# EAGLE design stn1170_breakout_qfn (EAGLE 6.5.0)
DESCRIPTION: Breakout Board; HW_REV: 1.1; PCB_REV: B; TITLE: STN1170 - Breakout Board

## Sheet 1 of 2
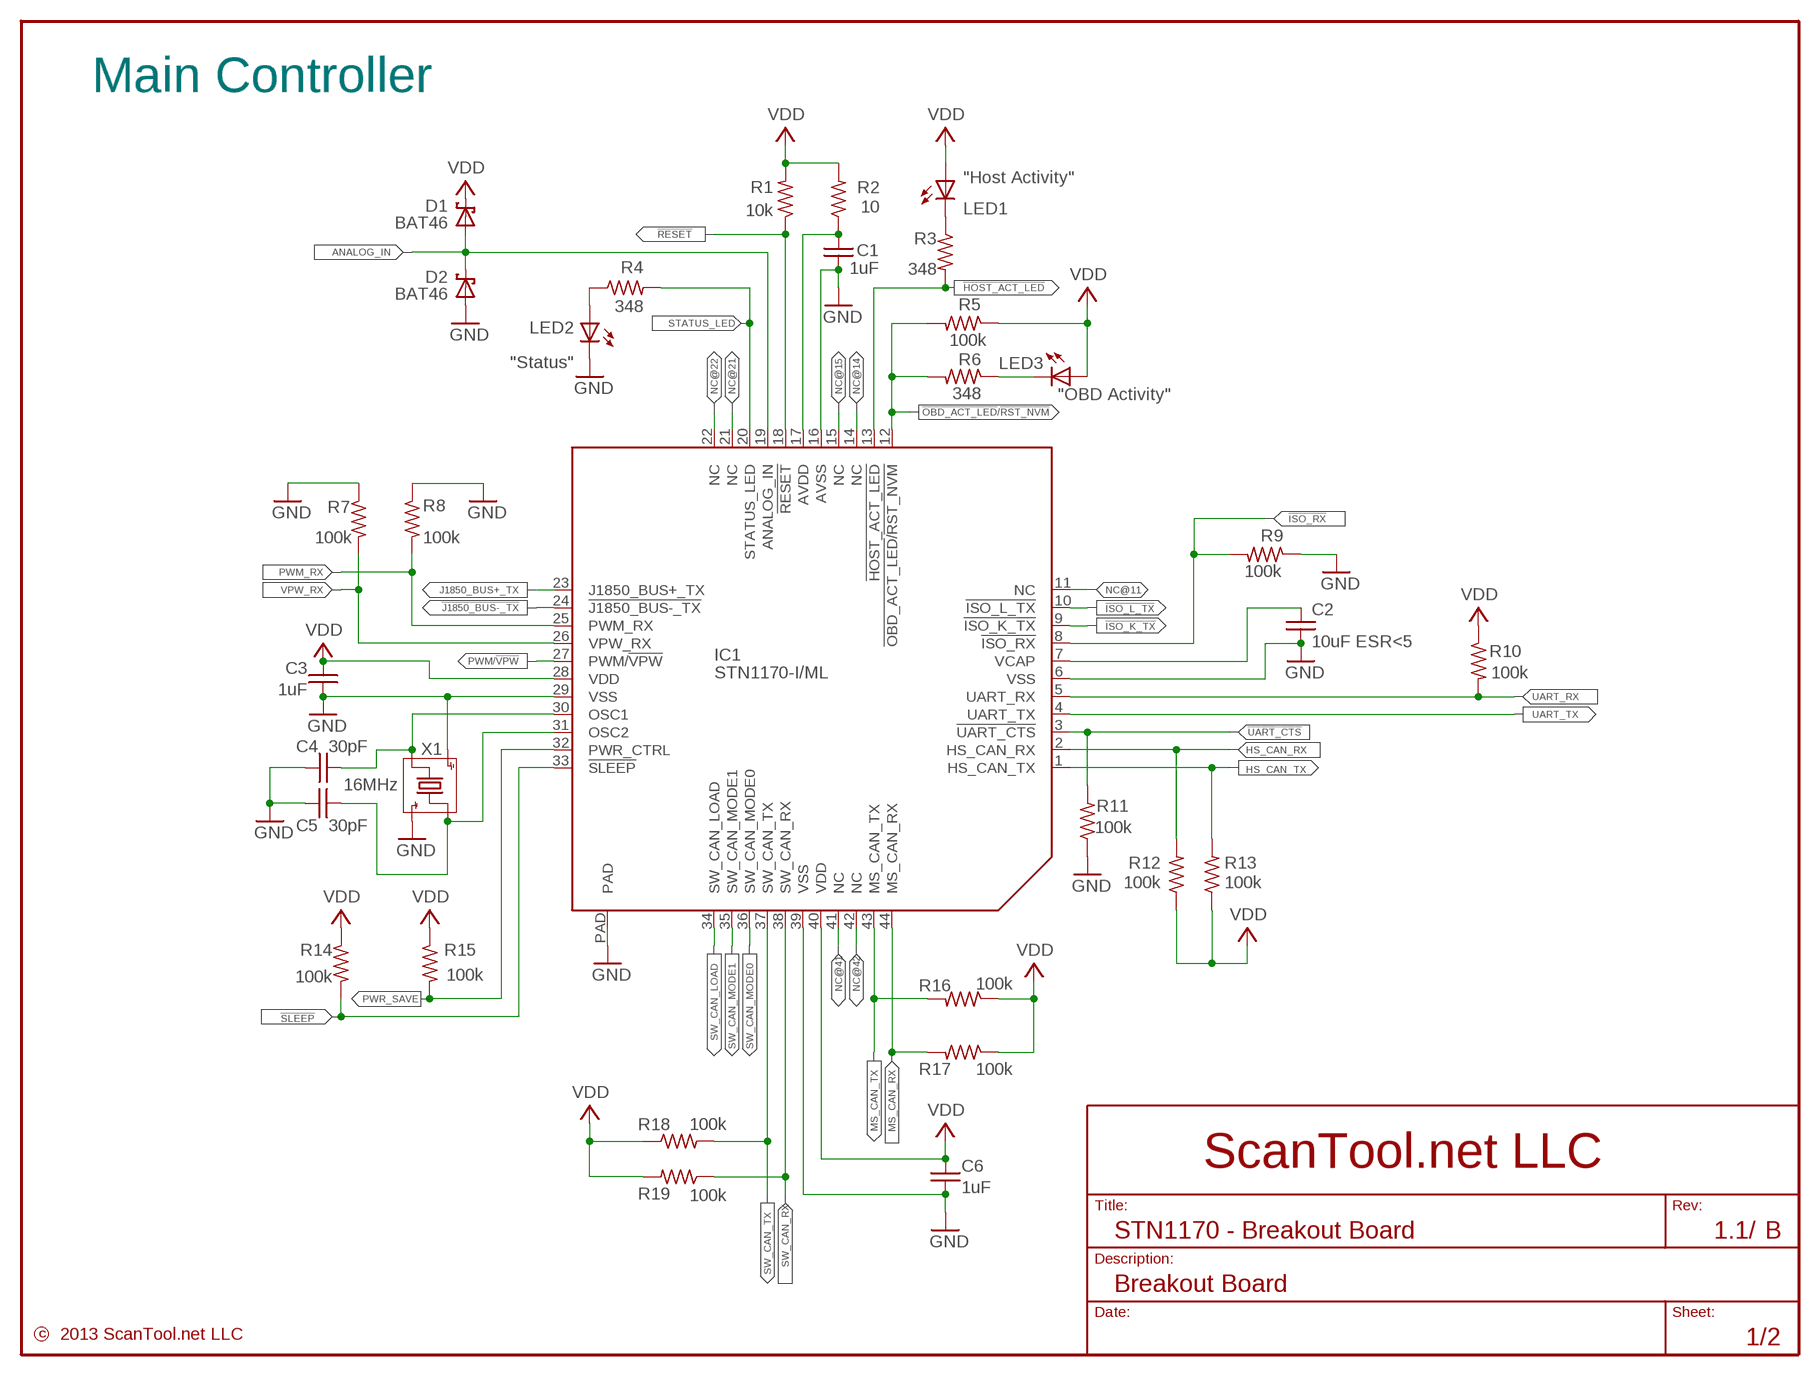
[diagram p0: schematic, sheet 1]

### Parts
C1  1uF  C-US_0603  [0603]
C2  10uF ESR<5  C-US_0805  [0805]
C3  1uF  C-US_0603  [0603]
C4  30pF  C-US_0603  [0603]
C5  30pF  C-US_0603  [0603]
C6  1uF  C-US_0603  [0603]
D1  BAT46  BAT46JFILM  [SOD-323_SCHOTTKY]
D2  BAT46  BAT46JFILM  [SOD-323_SCHOTTKY]
IC1  STN1170-I/ML  [QFN-44]
LED1  "Host Activity"  LED-0805  [0805-LED]
LED2  "Status"  LED-0805  [0805-LED]
LED3  "OBD Activity"  LED-0805  [0805-LED]
R1  10k  R-US_0603  [0603]
R2  10  R-US_0603  [0603]
R3  348  R-US_0603  [0603]
R4  348  R-US_0603  [0603]
R5  100k  R-US_0603  [0603]
R6  348  R-US_0603  [0603]
R7  100k  R-US_0603  [0603]
R8  100k  R-US_0603  [0603]
R9  100k  R-US_0603  [0603]
R10  100k  R-US_0603  [0603]
R11  100k  R-US_0603  [0603]
R12  100k  R-US_0603  [0603]
R13  100k  R-US_0603  [0603]
R14  100k  R-US_0603  [0603]
R15  100k  R-US_0603  [0603]
R16  100k  R-US_0603  [0603]
R17  100k  R-US_0603  [0603]
R18  100k  R-US_0603  [0603]
R19  100k  R-US_0603  [0603]
X1  16MHz  CRYSTAL-4PIN_NX3225SA  [3.2X2.5-MM]

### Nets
!HOST_ACT_LED: IC1.13(!HOST_ACT_LED) R3.2 ; also sheet 2
!ISO_K_TX: IC1.9(!ISO_K_TX) ; also sheet 2
!ISO_L_TX: IC1.10(!ISO_L_TX) ; also sheet 2
!ISO_RX: IC1.8(!ISO_RX) R9.2 ; also sheet 2
!J1850_BUS-_TX: IC1.24(!J1850_BUS-_TX) ; also sheet 2
!OBD_ACT_LED!/!RST_NVM: IC1.12(!OBD_ACT_LED!/!RST_NVM) R5.2 R6.2 ; also sheet 2
!RESET: IC1.18(!RESET) R1.1 ; also sheet 2
!SLEEP: IC1.33(!SLEEP) R14.2 ; also sheet 2
!UART_CTS: IC1.3(!UART_CTS) R11.2 ; also sheet 2
ANALOG_IN: D1.A D2.C IC1.19(ANALOG_IN) ; also sheet 2
AVDD [Supply]: C1.1 IC1.17(AVDD) R2.1
GND [Supply]: C1.2 C2.2 C3.1 C4.2 C5.2 C6.2 D2.A IC1.6(VSS) IC1.16(AVSS) IC1.29(VSS) IC1.39(VSS) IC1.PAD LED2.C R7.1 R8.1 R9.1 R11.1 X1.2(GND) X1.4(GND) ; also sheet 2
HS_CAN_RX: IC1.2(HS_CAN_RX) R12.2 ; also sheet 2
HS_CAN_TX: IC1.1(HS_CAN_TX) R13.2 ; also sheet 2
J1850_BUS+_TX: IC1.23(J1850_BUS+_TX) ; also sheet 2
MS_CAN_RX: IC1.44(MS_CAN_RX) R17.2 ; also sheet 2
MS_CAN_TX: IC1.43(MS_CAN_TX) R16.2 ; also sheet 2
N$1: LED1.C R3.1
N$2: LED3.C R6.1
N$3: C5.1 IC1.31(OSC2) X1.1(OSCX)
N$4: LED2.A R4.1
N$6: C4.1 IC1.30(OSC1) X1.3(OSCX)
NC@11: IC1.11(NC) ; also sheet 2
NC@14: IC1.14(NC) ; also sheet 2
NC@15: IC1.15(NC) ; also sheet 2
NC@21: IC1.21(NC) ; also sheet 2
NC@22: IC1.22(NC) ; also sheet 2
NC@41: IC1.41(NC) ; also sheet 2
NC@42: IC1.42(NC) ; also sheet 2
PWM/!VPW: IC1.27(PWM/!VPW) ; also sheet 2
PWM_RX: IC1.25(PWM_RX) R8.2 ; also sheet 2
PWR_SAVE: IC1.32(PWR_CTRL) R15.2 ; also sheet 2
STATUS_LED: IC1.20(STATUS_LED) R4.2 ; also sheet 2
STN1170_VCAP: C2.1 IC1.7(VCAP)
SW_CAN_LOAD: IC1.34(SW_CAN_LOAD) ; also sheet 2
SW_CAN_MODE0: IC1.36(SW_CAN_MODE0) ; also sheet 2
SW_CAN_MODE1: IC1.35(SW_CAN_MODE1) ; also sheet 2
SW_CAN_RX: IC1.38(SW_CAN_RX) R19.1 ; also sheet 2
SW_CAN_TX: IC1.37(SW_CAN_TX) R18.2 ; also sheet 2
UART_RX: IC1.5(UART_RX) R10.2 ; also sheet 2
UART_TX: IC1.4(UART_TX) ; also sheet 2
VDD [Supply]: C3.2 C6.1 D1.C IC1.28(VDD) IC1.40(VDD) LED1.A LED3.A R1.2 R2.2 R5.1 R10.1 R12.1 R13.1 R14.1 R15.1 R16.1 R17.1 R18.1 R19.2 ; also sheet 2
VPW_RX: IC1.26(VPW_RX) R7.2 ; also sheet 2

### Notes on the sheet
- Main Controller
- BAT46
- BAT46

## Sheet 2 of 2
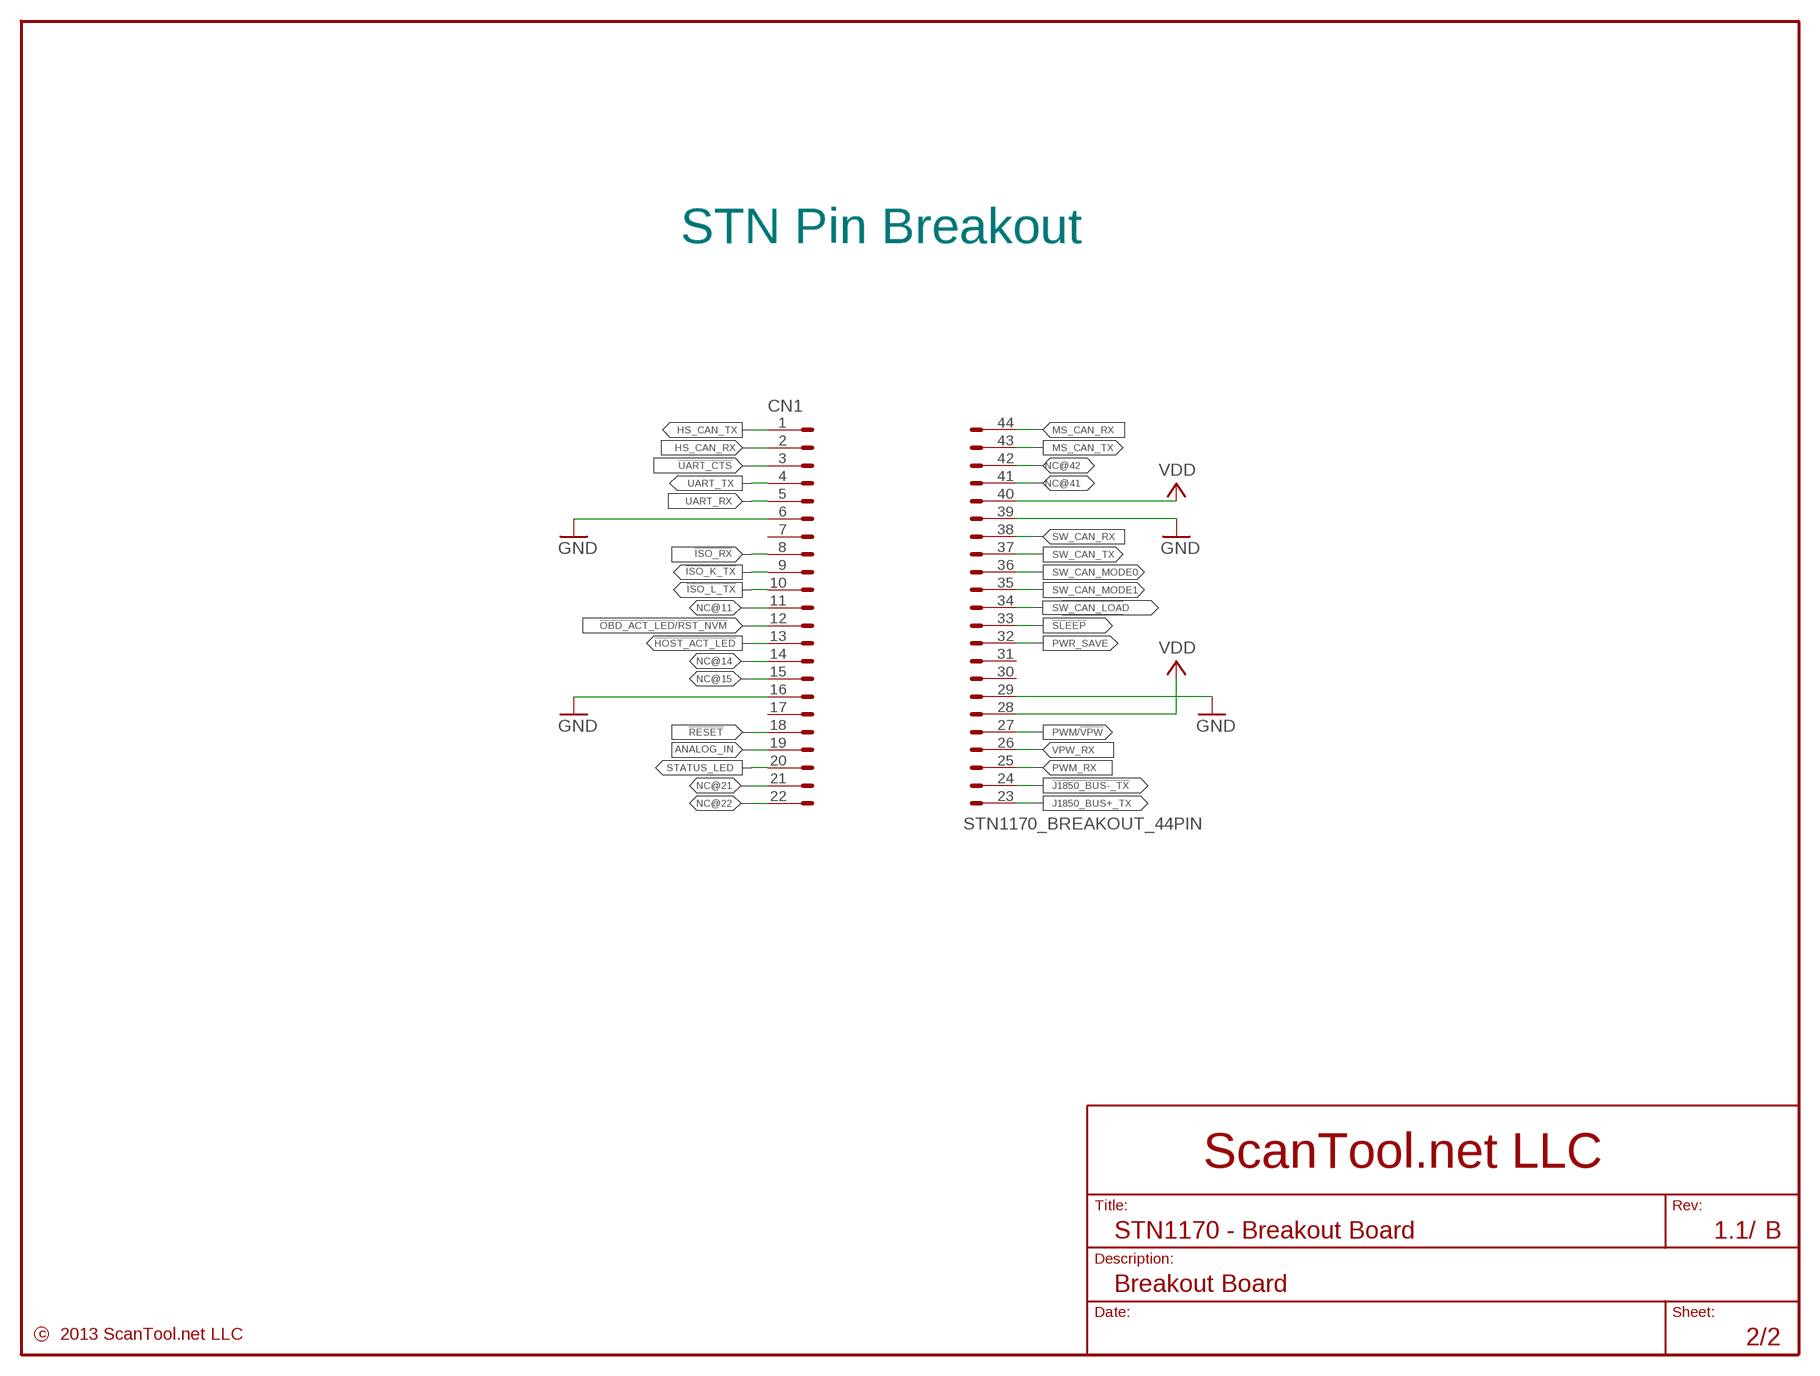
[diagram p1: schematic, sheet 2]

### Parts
CN1  STN1170_BREAKOUT_44PIN  [STN1170_BREAKOUT_44PIN]

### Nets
!HOST_ACT_LED: CN1.13 ; also sheet 1
!ISO_K_TX: CN1.9 ; also sheet 1
!ISO_L_TX: CN1.10 ; also sheet 1
!ISO_RX: CN1.8 ; also sheet 1
!J1850_BUS-_TX: CN1.24 ; also sheet 1
!OBD_ACT_LED!/!RST_NVM: CN1.12 ; also sheet 1
!RESET: CN1.18 ; also sheet 1
!SLEEP: CN1.33 ; also sheet 1
!UART_CTS: CN1.3 ; also sheet 1
ANALOG_IN: CN1.19 ; also sheet 1
GND [Supply]: CN1.6 CN1.16 CN1.29 CN1.39 ; also sheet 1
HS_CAN_RX: CN1.2 ; also sheet 1
HS_CAN_TX: CN1.1 ; also sheet 1
J1850_BUS+_TX: CN1.23 ; also sheet 1
MS_CAN_RX: CN1.44 ; also sheet 1
MS_CAN_TX: CN1.43 ; also sheet 1
NC@11: CN1.11 ; also sheet 1
NC@14: CN1.14 ; also sheet 1
NC@15: CN1.15 ; also sheet 1
NC@21: CN1.21 ; also sheet 1
NC@22: CN1.22 ; also sheet 1
NC@41: CN1.41 ; also sheet 1
NC@42: CN1.42 ; also sheet 1
PWM/!VPW: CN1.27 ; also sheet 1
PWM_RX: CN1.25 ; also sheet 1
PWR_SAVE: CN1.32 ; also sheet 1
STATUS_LED: CN1.20 ; also sheet 1
SW_CAN_LOAD: CN1.34 ; also sheet 1
SW_CAN_MODE0: CN1.36 ; also sheet 1
SW_CAN_MODE1: CN1.35 ; also sheet 1
SW_CAN_RX: CN1.38 ; also sheet 1
SW_CAN_TX: CN1.37 ; also sheet 1
UART_RX: CN1.5 ; also sheet 1
UART_TX: CN1.4 ; also sheet 1
VDD [Supply]: CN1.28 CN1.40 ; also sheet 1
VPW_RX: CN1.26 ; also sheet 1
Unconnected: CN1.7 CN1.17 CN1.30 CN1.31

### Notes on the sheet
- STN Pin Breakout

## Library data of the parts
C1-C6 = _stn_rcl:C-US: Capacitor, US Symbol; DESC: Capacitor; VALSTAT: VAL
CN1 = _stn_connector:STN1170_BREAKOUT_44PIN: STN1170-BREAKOUT BOARD, Male, 22X2, .0.01" Pitch Based on 2 Standard 22X1 .01" pitch male headers. Change Log DateAuthorChange July 05, 2012dduggan@scantool.netDevice created.; DESC: Header; PARTNUM: 0.1" male header; VALSTAT: PARTNUM
D1 D2 = _stn_diode:BAT46?FILM: BAT46 Schottky Diode; DESC: Diode, Schottky; MANUF: STMicroelectronics; PARTNUM: BAT46JFILM; SUPPLIER: Digikey:497-6653-1-ND; VALSTAT: PARTNUM
IC1 = _stn_scantool:STN1170: STN1170 Change Log DateAuthorChange July 12, 2012jason@scantool.netAdded attributes to device July 11, 2012vitaliy@scantool.netRenamed SW_CAN_HS_MODE pin to SW_CAN_LOAD April 11, 2012vit@scantool.netChanged UART_CTS pin polarity. Renamed OSCI/OSCOpins to OSC1/OSC2. April 10,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; DESC: IC, OBD-to-UART; MANUF: ScanTool.net, LLC; PARTNUM: ???; VALSTAT: VALUE
LED1-LED3 = _stn_led:LED: Light Emitting Diode; DESC: LED; VALSTAT: LABEL
R1-R19 = _stn_rcl:R-US: Resistor, US Symbol; DESC: Resistor; VALSTAT: VAL
X1 = _stn_crystal:CRYSTAL-4PIN: Crystal, 4 PIN March 16, 2010 vitaliy@scantool.netFixed pin assignments, verified package. March 4, 2010 jason@scantool.netCreated device from the NDK NX3225SA datasheet.; DESC: Crystal; MANUF: TXC; PARTNUM: 7M; VALSTAT: VAL

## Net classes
0 default: width 0.203 mm, drill 0.406 mm, clearance 0.203 mm
1 Supply: width 0.305 mm, drill 0.508 mm, clearance 0.254 mm
2 Vbat: width 0.61 mm, drill 0.813 mm, clearance 0.381 mm

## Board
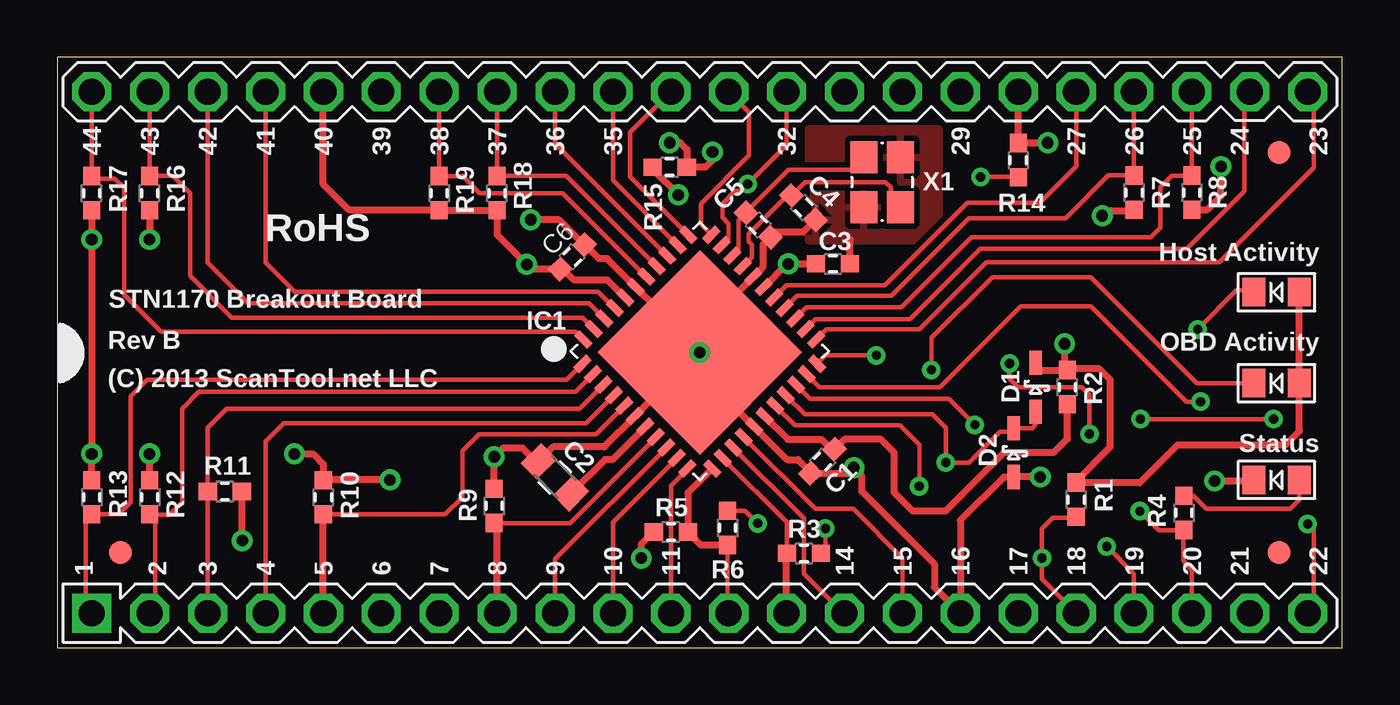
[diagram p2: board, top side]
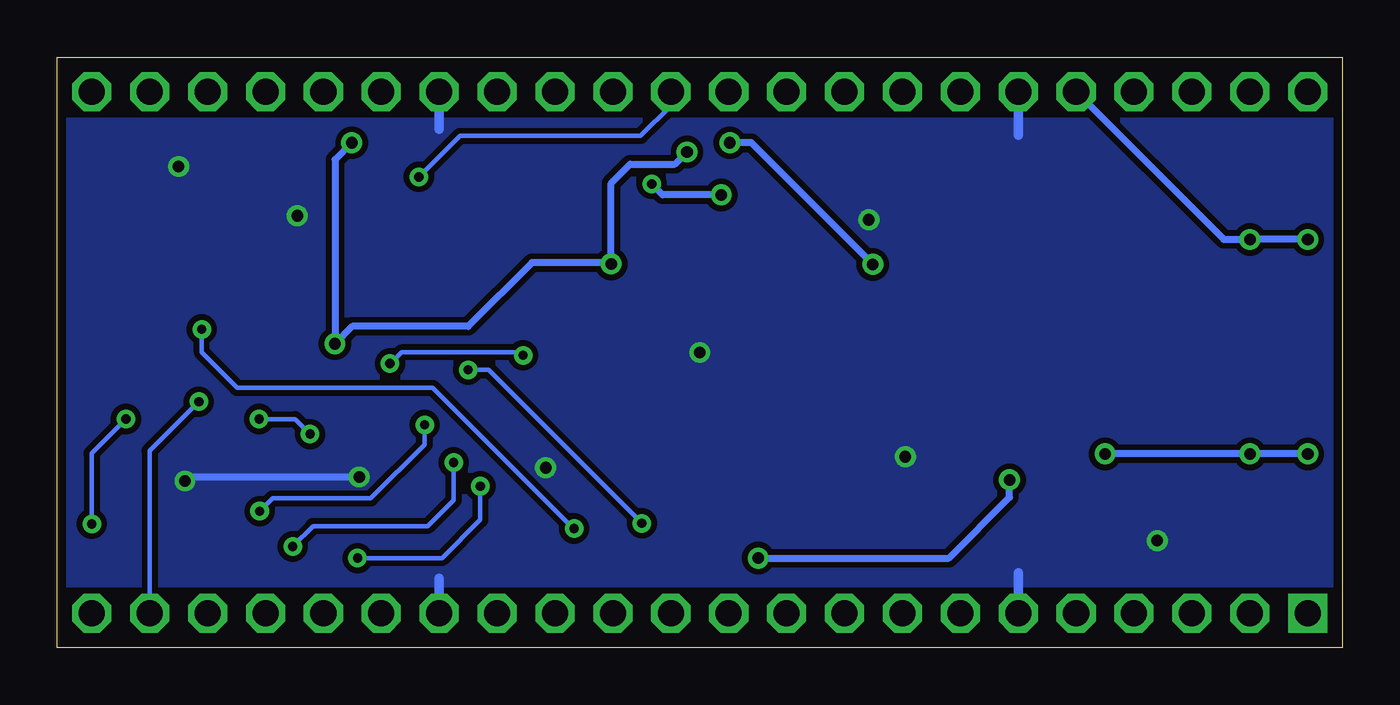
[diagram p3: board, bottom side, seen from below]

Size 56.39 x 25.91 mm. Coordinates in mm from the lower left corner, seen from the top.
Outline: 56.39,0 56.39,25.91 0,25.91 0,0 56.39,0
Copper layers (1*16): Top 0.035mm / dielectric 1.5mm / Bottom 0.035mm
Design rules "default": minimum track width 8mil, minimum drill 15mil, track to track 8mil, track to pad 8mil, pad to pad 8mil, via to via 8mil, smd to smd 8mil, copper to edge 15mil, drill to drill 8mil, minimum pad ring 10mil, minimum via ring 8mil, stop-mask expansion 4mil, vias tented up to drill 20mil, thermal gap 10mil

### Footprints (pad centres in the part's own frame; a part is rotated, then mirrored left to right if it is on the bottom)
0603 = smd 0.8 x 0.75: 1 -0.75,0; 2 0.75,0
0805 = smd 1 x 1.25: 1 -1,0; 2 1,0
STN1170_BREAKOUT_44PIN = drill 1.143 square: 1 -11.43,26.67 | drill 1.143 octagon: 2 -11.43,24.13; 3 -11.43,21.59; 4 -11.43,19.05; 5 -11.43,16.51; 6 -11.43,13.97; 7 -11.43,11.43; 8 -11.43,8.89; 9 -11.43,6.35; 10 -11.43,3.81; 11 -11.43,1.27; 12 -11.43,-1.27; 13 -11.43,-3.81; 14 -11.43,-6.35; 15 -11.43,-8.89; 16 -11.43,-11.43; 17 -11.43,-13.97; 18 -11.43,-16.51; 19 -11.43,-19.05; 20 -11.43,-21.59; 21 -11.43,-24.13; 22 -11.43,-26.67; 23 11.43,-26.67; 24 11.43,-24.13; 25 11.43,-21.59; 26 11.43,-19.05; 27 11.43,-16.51; 28 11.43,-13.97; 29 11.43,-11.43; 30 11.43,-8.89; 31 11.43,-6.35; 32 11.43,-3.81; 33 11.43,-1.27; 34 11.43,1.27; 35 11.43,3.81; 36 11.43,6.35; 37 11.43,8.89; 38 11.43,11.43; 39 11.43,13.97; 40 11.43,16.51; 41 11.43,19.05; 42 11.43,21.59; 43 11.43,24.13; 44 11.43,26.67
SOD-323_SCHOTTKY = smd 1.06 x 0.54: A 1.07,0; C -1.07,0
FIDUCIAL_40X100 = smd 1.016 x 1.016: P$1 0,0
QFN-44 = smd 0.8 x 0.35: 1 -3.988,3.287; 2 -3.988,2.637; 3 -3.988,1.987; 4 -3.988,1.337; 5 -3.988,0.687; 6 -3.988,0.037; 7 -3.988,-0.613; 8 -3.988,-1.263; 9 -3.988,-1.913; 10 -3.988,-2.563; 11 -3.988,-3.213; 23 4.012,-3.213; 24 4.012,-2.563; 25 4.012,-1.913; 26 4.012,-1.263; 27 4.012,-0.613; 28 4.012,0.037; 29 4.012,0.687; 30 4.012,1.337; 31 4.012,1.987; 32 4.012,2.637; 33 4.012,3.287 | smd 0.35 x 0.8: 12 -3.213,-3.988; 13 -2.563,-3.988; 14 -1.913,-3.988; 15 -1.263,-3.988; 16 -0.613,-3.988; 17 0.037,-3.988; 18 0.687,-3.988; 19 1.337,-3.988; 20 1.987,-3.988; 21 2.637,-3.988; 22 3.287,-3.988; 34 3.287,4.012; 35 2.637,4.012; 36 1.987,4.012; 37 1.337,4.012; 38 0.687,4.012; 39 0.037,4.012; 40 -0.613,4.012; 41 -1.263,4.012; 42 -1.913,4.012; 43 -2.563,4.012; 44 -3.213,4.012 | smd 6.35 x 6.35: PAD 0,0
0805-LED = smd 1 x 1.25: A 1,0; C -1,0
3.2X2.5-MM = smd 1.4 x 1.2: 1 -1.1,-0.8; 2 1.1,-0.8; 3 1.1,0.8; 4 -1.1,0.8

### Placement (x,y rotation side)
C1  33.58,8.18 225 top
C2  21.84,7.48 135 top
C3  34.04,16.84 180 top
C4  32.75,19.31 315 top
C5  30.76,18.54 315 top
C6  22.6,17.14 45 top
CN1  28.19,12.95 90 top
D1  42.93,11.43 270 top
D2  41.96,8.56 270 top
E$4  [FIDUCIAL_40X100]  53.59,21.72 0 top
E$5  [FIDUCIAL_40X100]  2.79,4.19 0 top
E$6  [FIDUCIAL_40X100]  53.59,4.19 180 top
IC1  28.19,12.95 45 top
LED1  53.49,15.6 0 top
LED2  53.49,7.37 0 top
LED3  53.49,11.61 0 top
R1  44.7,6.5 90 top
R2  44.32,11.43 90 top
R3  32.77,4.14 180 top
R4  49.43,5.92 270 top
R5  26.92,5.08 0 top
R6  29.41,5.26 270 top
R7  47.24,19.96 90 top
R8  49.78,19.96 90 top
R9  19.18,6.22 270 top
R10  11.68,6.6 270 top
R11  7.37,6.86 180 top
R12  4.06,6.6 270 top
R13  1.52,6.6 270 top
R14  42.16,21.39 270 top
R15  26.87,21.08 180 top
R16  4.06,19.94 90 top
R17  1.52,19.94 90 top
R18  19.3,19.94 90 top
R19  16.76,19.94 270 top
X1  36.2,20.42 270 top

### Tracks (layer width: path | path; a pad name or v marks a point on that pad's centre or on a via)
!HOST_ACT_LED
  Top 0.203: R3.2 32.02,5.51 IC1.13
  Top 0.305: CN1.13 32,4.13 R3.2
!ISO_K_TX
  Top 0.203: IC1.9 21.84,3.9 CN1.9
!ISO_L_TX
  Top 0.203: IC1.10 24.38,5.51 CN1.10
!ISO_RX
  Top 0.203: IC1.8 22.5,5.47 R9.2
  Top 0.305: CN1.8 19.3,5.35 R9.2
!J1850_BUS-_TX
  Top 0.203: IC1.24 33.27,14.4 37.41,14.4 40.51,17.5 49.55,17.5 52.07,20.02 52.07,24.13 CN1.24
!OBD_ACT_LED!/!RST_NVM
  Top 0.203: R6.2 29.41,1.57 CN1.12
  Top 0.305: IC1.12 27.67,6.79 R5.2 28.25,4.51 R6.2
!RESET  (via drill 0.41)
  Top 0.203: R1.1 44.67,5.71 43.69,5.71 43.2,5.23 v43.2,3.94 43.2,3.02 CN1.18 | IC1.18 32.37,9.75 36.98,9.75 37.82,8.91 v37.82,7.09
  Bottom 0.203: v37.82,7.09 37.82,5.61 39.5,3.94 v43.2,3.94
!SLEEP  (via drill 0.41)
  Top 0.203: R14.2 v40.51,20.65 | IC1.33 28.25,18.58 28.25,19.48 30.35,21.59 30.35,23.5 CN1.33 29.48,24.38
  Bottom 0.203: v40.51,20.65 38.71,22.45 30.79,22.45 29.46,23.77 CN1.33
!UART_CTS
  Top 0.203: IC1.3 22.92,10.49 7.44,10.49 6.6,9.65 6.6,6.87 | 6.6,6.87 R11.2 | 6.6,6.87 CN1.3
ANALOG_IN  (via drill 0.41)
  Top 0.203: IC1.19 32.8,10.24 38.41,10.24 38.99,9.65 v38.99,8.13 40.01,8.13 41.35,9.47 41.8,9.47 D2.C 42.78,9.63 42.93,9.78 D1.A | CN1.19 47.24,3.25 v46.05,4.45
  Bottom 0.203: v38.99,8.13 38.99,6.48 40.13,5.33 45.16,5.33 v46.05,4.45
AVDD
  Top 0.305: IC1.17 32.06,9.14 33.53,9.14 33.96,8.71 C1.1 34.54,9.14 36.14,9.14 36.73,8.56 36.73,6.81 37.54,5.99 38.96,5.99 41.53,8.56 43.71,8.56 44.32,9.17 R2.1
GND  (via drill 0.51)
  Top 0.305: X1.4 36.99,21.73 | v43.13,7.49 41.99,7.49 41.98,7.49 D2.A 41.53,7.49 39.62,5.59 CN1.16 | v20.78,18.77 22.02,18.77 C6.2 23.17,17.67 23.77,17.07 24.13,17.07 IC1.39 26.29,14.91 | v45.85,18.95 46,18.95 46.23,19.18 47.21,19.18 R7.1 | C4.2 32.74,18.24 31.52,18.24 C5.2 30.99,17.71 30.99,16.72 IC1.29 28.19,13.93 IC1.PAD | X1.2 | 39.62,1.65 CN1.16 | CN1.16 38.48,2.67 38.48,3.68 35.31,6.86 35.31,7.54 34.98,7.87 34.75,7.65 C1.2 33.05,7.72 32.51,8.26 32.03,8.26 IC1.16 29.59,10.69 | LED2.C 52.44,7.32 v50.77,7.32 | R8.1 50.46,19.21 51.05,19.81 v51.05,21.11 | C3.1 34.79,17.89 34.8,17.91 | R9.1 v19.18,8.38 19.56,8.76 20.42,8.76 21.13,8.05 C2.2 21.76,8.81 24,8.81 IC1.6 26.11,10.92 | v8.13,4.7 8.13,6.85 R11.1
  Bottom 0.305: v50.77,7.32 50.6,7.49 v43.13,7.49
  Bottom 0.406: CN1.6 14.22,3.3 | CN1.39 14.22,22.48 | CN1.29 39.62,22.73 | CN1.16 39.62,3.05
  other vias: 34.95,7.9 28.19,12.95
  pour Top: 32.97,22.78 38.68,22.78 38.68,17.83 32.97,17.83
  pour Bottom: 0.2,2.79 56.21,2.79 56.21,23.11 0.2,23.11
HS_CAN_RX
  Top 0.203: CN1.2 4.32,1.78 4.32,5.59 R12.2 4.08,5.84 4.95,5.84 5.49,6.38 5.49,10.49 6.22,11.23 22.74,11.23 IC1.2
HS_CAN_TX
  Top 0.203: IC1.1 22.35,11.76 3.96,11.76 3.23,11.02 3.23,6.38 2.7,5.85 R13.2 1.27,5.59 1.27,1.78 CN1.1
J1850_BUS+_TX
  Top 0.203: IC1.23 33.75,13.97 37.82,13.97 40.77,16.92 50.98,16.92 55.12,21.06 55.12,24.13 CN1.23
MS_CAN_RX
  Top 0.203: R17.2 | IC1.44 22.74,13.87 4.57,13.87 2.95,15.49 2.95,20.17 2.54,20.57 1.64,20.57 R17.2 | R17.2 CN1.44
MS_CAN_TX
  Top 0.203: 4.08,20.7 R16.2 | IC1.43 23.05,14.48 7.67,14.48 5.84,16.31 5.84,19.94 5.08,20.7 4.08,20.7 | 4.08,20.7 4.08,24.37 CN1.43
N$1  (via drill 0.41)
  Top 0.203: LED1.C 52.47,15.57 52.37,15.67 51.74,15.67 v50.04,13.97 | R3.1 33.71,4.14 v33.71,5.23
  Bottom 0.203: v33.71,5.23 33.73,5.23 39.9,11.4 48.49,11.4 50.04,12.95 v50.04,13.97
N$2  (via drill 0.41)
  Top 0.203: LED3.C 49.99,11.61 45.34,16.26 41.02,16.26 38.35,13.59 v38.35,12.19 | v30.73,5.46 30.19,6.01 R6.1
  Bottom 0.203: v30.73,5.46 37.47,12.19 v38.35,12.19
N$3
  Top 0.203: 35.36,21.49 X1.1 34.83,20.95 32.08,20.95 30.23,19.1 C5.1 30.23,19.05 29.9,18.72 29.9,17.47 IC1.31
N$4
  Top 0.203: R4.1 49.85,6.67 50.42,6.1 54.1,6.1 54.49,6.49 LED2.A
N$6
  Top 0.203: IC1.30 30.48,17.13 30.48,17.68 30.33,17.83 30.33,18.14 32.03,19.84 C4.1 32.8,20.42 36.35,20.42 36.58,20.19 36.58,19.74 X1.3 36.98,19.33
NC@11
  Top 0.203: IC1.11 27.65,7.83 26.92,7.11 CN1.11
NC@14
  Top 0.203: CN1.14 34.52,1.5 32.77,3.25 32.77,5.68 IC1.14
NC@15
  Top 0.203: IC1.15 33.27,6.1 34.92,6.1 37.08,3.94 CN1.15
NC@21  (via drill 0.41)
  Top 0.203: IC1.21 33.45,11.43 38.73,11.43 42.29,14.99 45.34,14.99 49.53,10.79 v50.16,10.79
  Bottom 0.203: v50.16,10.79 52.32,8.64 CN1.21
NC@22  (via drill 0.41)
  Top 0.203: v53.37,10.03 v47.52,10.03 | IC1.22 33.71,12.83 v35.94,12.83 | v54.86,5.44 55.12,5.18 55.12,1.78 CN1.22 | v45.29,9.37 45.29,11.1 44.96,11.43 42.16,11.43 41.78,11.81 v41.78,12.47
  Bottom 0.203: v53.37,10.03 54.87,8.53 v54.87,5.44 arc-90 v54.86,5.44 | v47.52,10.03 45.95,10.03 v45.29,9.37 | v41.78,12.47 41.76,12.47 41.27,12.95 36.07,12.95 v35.94,12.83
NC@41
  Top 0.203: CN1.41 9.14,16.89 10.41,15.62 23.74,15.62 IC1.41
NC@42
  Top 0.203: CN1.42 6.6,16.89 8.38,15.11 23.33,15.11 IC1.42
PWM/!VPW
  Top 0.203: IC1.27 32.01,15.9 36.32,15.9 39.93,19.51 43.1,19.51 44.7,21.11 CN1.27
PWM_RX
  Top 0.203: CN1.25 R8.2 48.9,20.7 48.39,20.19 48.39,18.41 47.98,18.01 40.11,18.01 37.03,14.94 32.88,14.94 IC1.25
PWR_SAVE  (via drill 0.41, 0.51)
  Top 0.203: CN1.32 32,22.05 v30.3,20.34 30,20.04 29.74,20.04 29.18,19.48 29.18,18.87 29.46,18.59 29.46,17.95 IC1.32
  Top 0.305: R15.2 26.12,20.99 v27.25,19.86
  Bottom 0.203: 30.28,20.37 v30.3,20.34
  Bottom 0.305: v27.25,19.86 29.82,19.86 v30.3,20.34
STATUS_LED  (via drill 0.41)
  Top 0.203: IC1.20 33.04,10.92 39.12,10.92 v40.26,9.78 | v47.5,5.99 48.32,5.17 R4.2 49.4,5.14 49.4,3.81 49.78,3.43 CN1.20
  Bottom 0.203: v47.5,5.99 46.94,6.55 42.62,6.55 40.26,8.91 v40.26,9.78
STN1170_VCAP
  Top 0.305: C2.1 24.03,8.26 24.36,8.26 IC1.7
SW_CAN_LOAD
  Top 0.203: IC1.34 25.15,20.65 25.15,22.61 CN1.34
SW_CAN_MODE0
  Top 0.203: IC1.36 21.84,22.11 CN1.36
SW_CAN_MODE1
  Top 0.203: CN1.35 24.38,20.49 IC1.35
SW_CAN_RX
  Top 0.203: IC1.38 22.18,19.94 18.54,19.94 17.78,20.7 17.77,20.69 R19.1 CN1.38
SW_CAN_TX
  Top 0.203: CN1.37 R18.2 19.32,20.7 22.34,20.7 IC1.37
UART_RX
  Top 0.203: 11.7,5.84 R10.2 17.03,5.85 17.78,6.6 17.78,8.64 18.52,9.37 23.64,9.37 IC1.5
  Top 0.305: CN1.5 R10.2
UART_TX
  Top 0.203: CN1.4 9.14,9.07 9.93,9.86 23.2,9.86 IC1.4
VDD  (via drill 0.51, 0.51 pad 0.41)
  Top 0.305: 42.22,22.15 42.09,22.15 | 42.22,22.15 42.2,22.14 R14.1 CN1.28 | R12.1 v4.06,8.51 | R16.1 v4.06,17.91 | CN1.40 11.68,20.32 12.81,19.19 R19.2 R18.1 19.3,18.11 v20.6,16.82 20.8,16.61 C6.1 22.2,16.61 22.68,16.13 24.15,16.13 IC1.40 | IC1.28 32.03,16.84 v32.08,16.84 C3.2 | 42.22,22.15 v43.46,22.15 | v26.87,22.15 27.33,22.15 27.64,21.84 27.64,21.09 R15.1 28.45,21.08 28.75,21.39 v28.75,21.74 | LED1.A LED3.A 54.49,9.51 53.87,8.89 49.15,8.89 47.5,7.24 44.72,7.24 R1.2 44.7,7.32 46.2,8.81 46.2,11.76 45.73,12.23 44.37,12.23 R2.2 | R5.1 25.63,4.54 v25.63,3.94 | R13.1 v1.52,8.51 v1.52,17.91 R17.1 | v10.41,8.51 11.23,8.51 11.68,8.05 R10.1 11.7,7.37 v14.61,7.37 | v44.2,13.34 44.2,12.31 R2.2 | D1.C 42.93,12.18 R2.2
  Bottom 0.305: CN1.40 5.21,17.91 v4.06,17.91 v1.52,17.91 | v20.6,16.82 25.93,22.15 v26.87,22.15 | v28.75,21.74 29.29,21.21 31.24,21.21 32.08,20.37 v32.08,16.84 32.13,16.89 35.56,16.89 38.35,14.1 43.43,14.1 v44.2,13.34 44.2,21.41 v43.46,22.15 | v1.52,8.51 v4.06,8.51 v10.41,8.51 | v25.63,3.94 17.27,3.94 14.61,6.6 v14.61,7.37
VPW_RX
  Top 0.203: CN1.26 R7.2 46.11,20.71 44.25,18.85 40.01,18.85 36.6,15.44 32.46,15.44 IC1.26

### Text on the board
tPlace: 44 | 43 | 42 | 41 | 40 | 39 | 38 | 37 | 36 | 35 | 32 | 29 | 27 | 26 | 25 | 24 | 23 | RoHS | Host Activity | STN1170 Breakout Board | OBD Activity | Rev B | (C) 2013 ScanTool.net LLC | Status | 1 | 2 | 3 | 4 | 5 | 6 | 7 | 8 | 9 | 10 | 11 | 14 | 15 | 16 | 17 | 18 | 19 | 20 | 21 | 22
